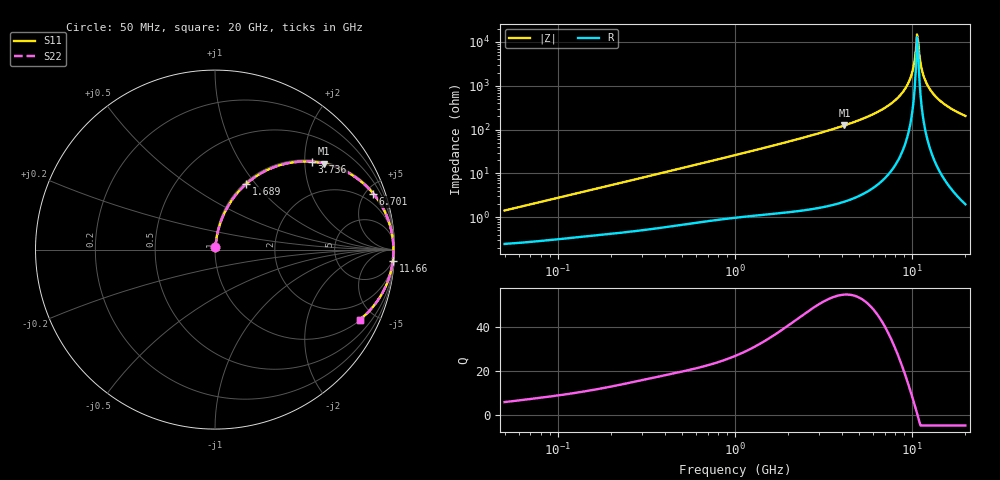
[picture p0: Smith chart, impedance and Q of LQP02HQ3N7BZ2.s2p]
!Murata Part Number: LQP02HQ3N7BZ2
!These Parameters are Measured in Series Mode Connection
!  o--[Z]--o
!Port1  Port2
!  o-------o
!Freq. Start=50[MHz] Stop=20[GHz], 401[Steps]
# Hz S RI R 50
!Freq.(Hz) S11(Real) S11(Imag) S21(Real) S21(Imag) S12(Real) S12(Imag) S22(Real) S22(Imag)
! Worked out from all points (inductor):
!   401 points, 50 MHz to 20 GHz, reference 50 ohm
!   read as one part in series: L = 4.45 nH near 51.52 MHz
!   highest Q = 54.9 at 4.149 GHz (marker M1), where L = 4.78 nH
!   self-resonance near 10.66 GHz
!   S11 on the Smith chart (normalised r, x): 50 MHz: 1.00, +0.03; 1.689 GHz: 1.02, +0.89; 3.736 GHz: 1.04, +2.17; 6.701 GHz: 1.13, +5.62; 11.66 GHz: 4, -32; 20 GHz: 1.04, -4.10
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5e7  0.00266 0.014  0.9973 -0.014  0.9973 -0.014  0.00266 0.014
1.364002e8  0.00494 0.0369  0.9951 -0.0369  0.9951 -0.0369  0.00494 0.0369
3.721004e8  0.0151 0.0967  0.9849 -0.0967  0.9849 -0.0967  0.0151 0.0967
1e9  0.0717 0.24  0.9283 -0.24  0.9283 -0.24  0.0717 0.24
1.689197e9  0.1718 0.3638  0.8282 -0.3638  0.8282 -0.3638  0.1718 0.3638
2.728004e9  0.3603 0.4699  0.6397 -0.4699  0.6397 -0.4699  0.3603 0.4699
3.736399e9  0.5406 0.4892  0.4594 -0.4892  0.4594 -0.4892  0.5406 0.4892
4.149438e9  0.6065 0.4795  0.3935 -0.4795  0.3935 -0.4795  0.6065 0.4795
6.701223e9  0.8819 0.3113  0.1181 -0.3113  0.1181 -0.3113  0.8819 0.3113
7.442007e9  0.9249 0.2501  0.0751 -0.2501  0.0751 -0.2501  0.9249 0.2501
8.516016e9  0.966 0.1625  0.034 -0.1625  0.034 -0.1625  0.966 0.1625
9.457416e9  0.9856 0.0895  0.0144 -0.0895  0.0144 -0.0895  0.9856 0.0895
1.004137e10  0.9918 0.0466  0.00819 -0.0466  0.00819 -0.0466  0.9918 0.0466
1.050288e10  0.9939 0.0142  0.00605 -0.0142  0.00605 -0.0142  0.9939 0.0142
1.066139e10  0.9942 0.00336  0.00581 -0.00336  0.00581 -0.00336  0.9942 0.00336
1.098561e10  0.994 -0.0183  0.00605 0.0183  0.00605 0.0183  0.994 -0.0183
1.131968e10  0.9928 -0.04  0.00723 0.04  0.00723 0.04  0.9928 -0.04
1.166392e10  0.9906 -0.0615  0.00937 0.0615  0.00937 0.0615  0.9906 -0.0615
1.257102e10  0.9812 -0.1149  0.0188 0.1149  0.0188 0.1149  0.9812 -0.1149
1.396067e10  0.9583 -0.1871  0.0417 0.1871  0.0417 0.1871  0.9583 -0.1871
1.646126e10  0.9012 -0.2909  0.0988 0.2909  0.0988 0.2909  0.9012 -0.2909
2e10  0.8056 -0.3909  0.1944 0.3909  0.1944 0.3909  0.8056 -0.3909
